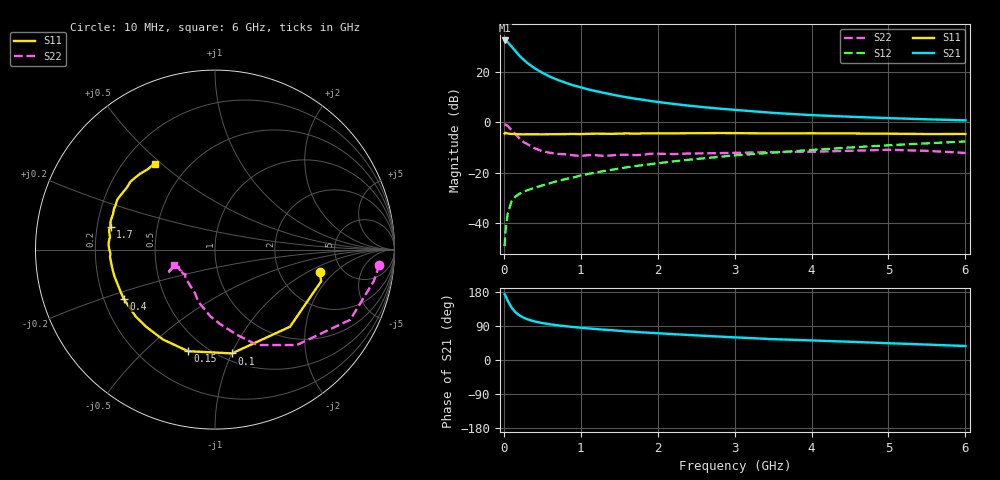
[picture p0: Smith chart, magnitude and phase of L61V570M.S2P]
!  INFINEON TECHNOLOGIES Small Signal Semiconductors
! BFR380L3 , Si-NPN RF-Transistor in TSLP-3-1
!  Vce=1.5 V,  Ic=70 mA
! Common Emitter S-Parameters:  07. March 2005
#  GHz  S  MA  R  50
! f  S11  S21  S12  S22
! GHz  Mag  Ang  Mag  Ang  Mag  Ang  Mag  Ang
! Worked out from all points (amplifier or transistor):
!   36 points, 10 MHz to 6 GHz, reference 50 ohm
!   highest |S21| = 32.4 dB at 10 MHz (marker M1)
!   |S21| within 3 dB of that: start of sweep to 116.8 MHz
!   unconditionally stable (mu >= 1): 1.177 GHz to 5.549 GHz
!   at 250 MHz: K = 0.52, MSG = 26.3 dB, |S12| = -27.7 dB
!   at 1.4 GHz: K = 1.03, MAG = 13.9 dB, |S12| = -18.8 dB
!   at 6 GHz: K = 0.99, MSG = 4.2 dB, |S12| = -7.6 dB
!   S11 on the Smith chart (normalised r, x): 10 MHz: 3.40, -1.35; 100 MHz: 0.57, -1.00; 150 MHz: 0.40, -0.69; 400 MHz: 0.28, -0.23; 1.7 GHz: 0.26, +0.10; 6 GHz: 0.33, +0.48
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0.01  0.598 -12.3  41.81 173.5  0.0035 70.8  0.9201 -5.2
0.02  0.6172 -16.6  41.25 170.6  0.0066 77.0  0.9022 -11.2
0.05  0.5993 -45.8  38.65 156.4  0.0154 71.3  0.8489 -27.4
0.1  0.586 -80.7  31.77 138.5  0.0271 58.3  0.7003 -49.4
0.15  0.5856 -104.9  25.72 126.1  0.0335 52.9  0.5816 -66.1
0.2  0.5788 -120.2  21.1 118.1  0.0382 50.6  0.4852 -76.2
0.25  0.5761 -131.8  17.76 112.4  0.0413 49.3  0.4114 -86.8
0.3  0.578 -139.8  15.18 107.9  0.0446 49.6  0.3726 -94.0
0.4  0.5782 -151.8  11.77 101.7  0.0503 50.8  0.3058 -107.5
0.5  0.5758 -159.2  9.572 97.5  0.0561 53.5  0.266 -115.0
0.6  0.5792 -164.6  8.002 94.2  0.062 55.6  0.2487 -122.1
0.7  0.5813 -168.4  6.922 91.5  0.0682 58.0  0.236 -129.0
0.9  0.5866 -176.1  5.414 87.1  0.0802 60.6  0.2212 -139.0
1.1  0.5898 179.5  4.477 83.3  0.0948 62.4  0.2233 -143.0
1.4  0.5888 173.2  3.554 78.8  0.1144 64.0  0.2203 -148.4
1.7  0.5952 168.0  2.949 74.4  0.1345 64.7  0.2232 -154.6
2.2  0.6015 160.8  2.315 68.2  0.1674 65.0  0.2337 -154.7
2.8  0.6117 152.9  1.865 61.8  0.2062 64.8  0.2445 -158.5
3.5  0.6003 144.8  1.534 55.0  0.2503 62.5  0.2564 -156.6
4.5  0.5999 138.5  1.286 48.1  0.316 60.6  0.272 -155.5
5.5  0.5841 130.2  1.144 40.7  0.3823 56.2  0.2715 -155.6
6  0.5858 125.1  1.091 36.9  0.4157 53.9  0.2464 -159.7
